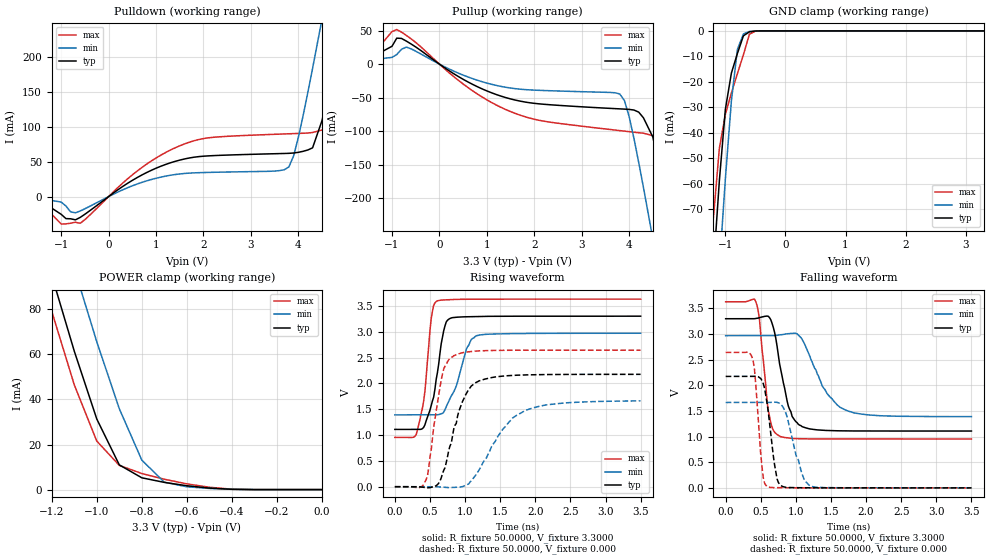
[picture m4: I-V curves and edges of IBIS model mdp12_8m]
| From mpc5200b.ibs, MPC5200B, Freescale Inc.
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|   Model mdp12_8m
[Model]   mdp12_8m
Model_type   I/O
Polarity   Non-Inverting
Enable   Active-High
Vinl =   0.8000V
Vinh =   2.0000V
Vmeas =   1.5000V
C_comp   2.1096pF   1.4802pF   2.7108pF
[Temperature Range]   27.0000   0.1250k   -40.0000
[Voltage Range]   3.3000V   2.9700V   3.6300V
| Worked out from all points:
|   slope of the pulldown table from 0 to 0.495 V, typ, clamps not added: 21.4 ohm
|   slope of the pullup table from 0 to 0.495 V, typ, clamps not added: 22 ohm
|   GND clamp passes 1 mA (typ) near -0.64 V on its own axis
|   POWER clamp passes 1 mA (typ) near -0.53 V on its own axis
|   rising waveform, R_fixture 50.0000, V_fixture 3.3000: 20-80 % time 160ps typ, 231ps min, 118ps max; typ from 1.11 V to 3.3 V
|   rising waveform, R_fixture 50.0000, V_fixture 0.000: 20-80 % time 268ps typ, 474ps min, 171ps max; typ from 0 V to 2.17 V
|   falling waveform, R_fixture 50.0000, V_fixture 3.3000: 20-80 % time 186ps typ, 358ps min, 116ps max; typ from 3.3 V to 1.11 V
|   falling waveform, R_fixture 50.0000, V_fixture 0.000: 20-80 % time 119ps typ, 190ps min, 85.9ps max; typ from 2.17 V to 0 V
[Pulldown]
| voltage   I(typ)   I(min)   I(max)
-3.3V     -1.242mA   -1.033mA   -1.021mA
-1.5V     -3.208mA   -2.394mA   -4.182mA
-1V       -25.48mA   -7.858mA   -39.49mA
-600mV    -29.97mA   -20.72mA   -38.34mA
1.4V      50.58mA    31.69mA    70.03mA
3.7V      61.96mA    38.47mA    90.02mA
3.9V      62.65mA    58.57mA    90.52mA
4.3V      70.11mA    184.4mA    92.13mA
4.5V      109.5mA    255.6mA    95.71mA
4.9V      248.4mA    401.7mA    125.6mA
5.3V      398mA      550.3mA    263.5mA
6.6V      902.3mA    1.042A     769.6mA
[Pullup]
| voltage   I(typ)   I(min)   I(max)
-3.3V     3.197mA    4.639mA    3.144mA
-1.5V     7.492mA    5.928mA    6.974mA
-900mV    38.83mA    14.34mA    51.69mA
-700mV    34.5mA     25.49mA    43.02mA
1.4V      -49.98mA   -34.56mA   -67.87mA
3.8V      -66.77mA   -44.54mA   -99.21mA
4V        -67.56mA   -78.63mA   -100.8mA
4.2V      -71.61mA   -146.6mA   -102.4mA
4.5V      -109.1mA   -261.6mA   -106.8mA
4.9V      -253.6mA   -421.6mA   -141.2mA
5.3V      -414.2mA   -584.5mA   -261.5mA
6.6V      -950.2mA   -1.121A    -794.4mA
[GND_clamp]
| voltage   I(typ)   I(min)   I(max)
-3.3V     -948.1mA   -982.8mA   -929.6mA
-1.3V     -130.7mA   -168mA     -108.8mA
-1.2V     -93.35mA   -129.8mA   -73.5mA
-1.1V     -58.65mA   -92.83mA   -45.99mA
-1V       -30.69mA   -57.94mA   -32.68mA
-900mV    -16.54mA   -27.44mA   -24.36mA
-800mV    -8.854mA   -7.262mA   -16.75mA
-700mV    -1.936mA   -1.183mA   -9.358mA
-600mV    -366uA     -212.8uA   -1.293mA
-500mV    -39.22uA   -34.56uA   -92.73uA
3.3V      541.3pA    33.88uA    287.7pA
[POWER_clamp]
| voltage   I(typ)   I(min)   I(max)
-3.3V     897.6mA    912.2mA    893.7mA
-1.3V     130.2mA    167.4mA    114.6mA
-1.2V     95.06mA    132.3mA    79.13mA
-1.1V     61.46mA    98.2mA     46.53mA
-1V       31.32mA    65.57mA    21.52mA
-900mV    10.96mA    35.88mA    10.75mA
-800mV    5.231mA    13.06mA    7.129mA
-700mV    3.197mA    3.28mA     4.595mA
-600mV    1.712mA    1.263mA    2.547mA
-500mV    672.1uA    514.1uA    1.035mA
-400mV    127.3uA    134.7uA    183.8uA
0V        541.3pA    4.807nA    325.5pA
[Ramp]
| variable   typ   min   max
dV/dt_r   1.2951/0.2640n   0.8376/0.3594n   1.5848/0.1664n
dV/dt_f   1.3135/0.1911n   0.8849/0.3102n   1.6058/0.1182n
R_load = 50.0000
[Rising Waveform]
R_fixture = 50.0000
V_fixture = 3.3000
V_fixture_min = 2.9700
V_fixture_max = 3.6300
| time   V(typ)   V(min)   V(max)
0s        1.109V     1.39V      953.6mV
303.6ps   1.109V     1.39V      1.006V
410.7ps   1.149V     1.391V     1.658V
517.9ps   1.569V     1.39V      3.249V
607.1ps   2.212V     1.392V     3.597V
732.1ps   3.189V     1.548V     3.618V
875ps     3.28V      1.949V     3.625V
1.018ns   3.289V     2.658V     3.628V
1.161ns   3.294V     2.921V     3.629V
3.5ns     3.3V       2.97V      3.63V
[Rising Waveform]
R_fixture = 50.0000
V_fixture = 0.000
| time   V(typ)   V(min)   V(max)
0s        47.04nV    148.4nV    115.8nV
446.4ps   -18.94mV   259.9uV    138.6mV
607.1ps   39.91mV    -2.322mV   1.622V
678.6ps   253.4mV    -7.857mV   2.18V
839.3ps   1.119V     -13.85mV   2.535V
964.3ps   1.652V     1.382mV    2.592V
1.125ns   1.99V      171.6mV    2.622V
1.518ns   2.138V     1.076V     2.639V
1.857ns   2.164V     1.472V     2.642V
3.5ns     2.175V     1.661V     2.642V
[Falling Waveform]
R_fixture = 50.0000
V_fixture = 3.3000
V_fixture_min = 2.9700
V_fixture_max = 3.6300
| time   V(typ)   V(min)   V(max)
0s        3.3V       2.97V      3.63V
428.6ps   3.304V     2.97V      3.634V
482.1ps   3.321V     2.97V      3.28V
607.1ps   3.348V     2.969V     1.511V
767.9ps   2.419V     2.985V     1.01V
946.4ps   1.394V     3.014V     965.3mV
1.107ns   1.185V     2.852V     956.9mV
1.375ns   1.125V     1.988V     954mV
1.714ns   1.111V     1.514V     953.6mV
3.5ns     1.109V     1.391V     953.6mV
[Falling Waveform]
R_fixture = 50.0000
V_fixture = 0.000
| time   V(typ)   V(min)   V(max)
0s        2.175V     1.666V     2.642V
375ps     2.175V     1.666V     2.554V
410.7ps   2.178V     1.666V     2.307V
517.9ps   2.092V     1.666V     405.7mV
589.3ps   1.656V     1.666V     25.18mV
732.1ps   174.9mV    1.668V     3.161mV
803.6ps   31.15mV    1.601V     2.09mV
1.089ns   2.305mV    266.6mV    250.1uV
1.196ns   1.341mV    43.22mV    116.7uV
3.5ns     326.6nV    2.946uV    -402.3nV
